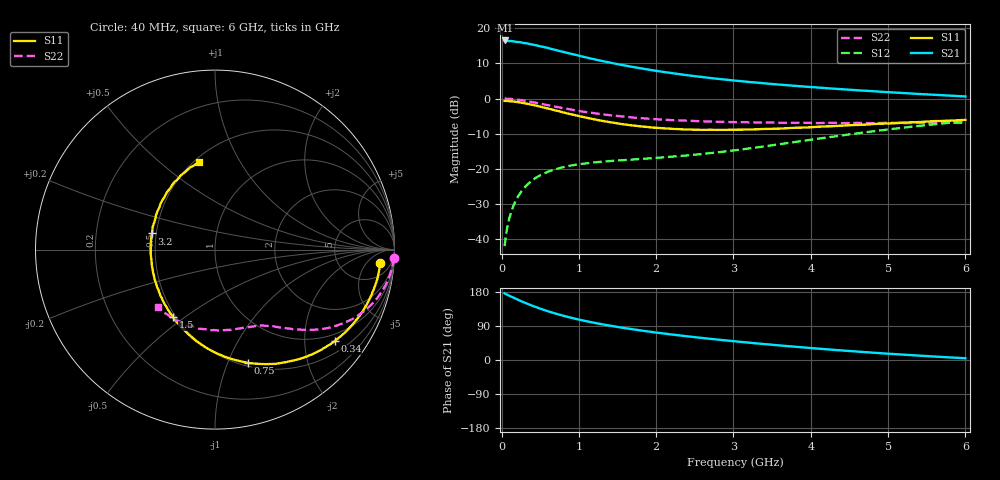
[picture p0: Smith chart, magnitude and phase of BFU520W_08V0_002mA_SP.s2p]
! Filename:  P:\Prog\Test\Noise\ATS_data\Testdata_Net\Run2\BFU520W_APM2013_06_A05_08p0V_002mA_SP_CM01_D.s2p
! Date/Time: Tue 26/Mar/2013 18:01:42
! BFU520W_APM2013_06_A05_08p0V_1to20mA_SP_CM01_Bias2_R.s2p
! MDIF S-parameter v. bias file
! BFU520W_APM2013_06_A05_08p0V_1to20mA_SP_CM01
! Date/time Thu Mar 21 15:28:29 2013
! VAR V_out= 8.0000
! VAR I_out= 2.0000
! VAR V_in= 0.8065
! VAR I_in= 0.0215
! Device data file deembeded for feedlines and parallel
! Original file: \Run2\BFU520W_APM2013_06_A05_08p0V_002mA_SP_CM01_R.s2p
! Feed-files: PR019V01_070313_Feed1.s2p, PR019V01_070313_Feed2.s2p
! Parallel-file: PR019V01_070313_Par.s2p
# MHz S MA R 50
!  Freq-MHz  S11-mag  S11-arg  S21-mag  S21-arg  S12-mag  S12-arg  S22-mag  S22-arg
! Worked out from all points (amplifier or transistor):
!   98 points, 40 MHz to 6 GHz, reference 50 ohm
!   highest |S21| = 16.5 dB at 50 MHz (marker M1)
!   |S21| within 3 dB of that: start of sweep to 750.4 MHz
!   unconditionally stable (mu >= 1): 2.391 GHz to 3.471 GHz
!   at 300 MHz: K = 0.18, MSG = 20.5 dB, |S12| = -25.2 dB
!   at 1.6 GHz: K = 0.78, MSG = 13.4 dB, |S12| = -17.5 dB
!   at 6 GHz: K = 0.82, MSG = 3.5 dB, |S12| = -6.5 dB
!   S11 on the Smith chart (normalised r, x): 40 MHz: 12, -13; 340 MHz: 0.79, -2.74; 750 MHz: 0.53, -1.18; 1.5 GHz: 0.48, -0.45; 3.2 GHz: 0.47, +0.10; 6 GHz: 0.53, +0.69
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40  0.9244 -4.6  6.654 176.0  0.00799 86.8  0.9968 -2.6
50  0.9233 -5.7  6.678 174.8  0.009908 86.3  0.9951 -3.2
90  0.9189 -10.3  6.546 170.7  0.01775 83.5  0.9912 -5.9
120  0.9124 -13.8  6.574 167.8  0.02349 81.4  0.986 -7.8
220  0.8853 -24.8  6.356 158.4  0.04164 75.0  0.9585 -13.9
340  0.8396 -37.5  6.038 147.9  0.06068 68.1  0.9138 -20.6
420  0.8038 -45.3  5.785 141.5  0.07162 64.1  0.8806 -24.4
550  0.7428 -57.5  5.375 132.0  0.08619 58.5  0.8241 -29.8
600  0.7213 -61.9  5.227 128.7  0.09104 56.6  0.8036 -31.6
750  0.6566 -73.9  4.728 119.6  0.1028 52.1  0.7461 -36.3
900  0.5973 -85.1  4.314 111.5  0.1118 48.7  0.697 -40.0
1050  0.5482 -95.3  3.933 104.5  0.1182 46.4  0.6524 -43.1
1250  0.4932 -107.7  3.508 96.2  0.1253 44.4  0.6079 -46.5
1500  0.4432 -121.8  3.079 87.2  0.1316 43.6  0.5642 -50.2
1800  0.4018 -137.3  2.686 78.0  0.1384 44.3  0.5258 -54.0
2050  0.3806 -149.1  2.424 71.2  0.1446 45.7  0.5042 -57.1
2500  0.3599 -168.7  2.079 60.2  0.1592 49.2  0.4792 -63.2
3100  0.3614 169.0  1.76 47.7  0.1889 54.3  0.4611 -72.4
3200  0.3624 165.6  1.719 45.8  0.1954 54.9  0.4583 -73.9
4100  0.3974 139.8  1.431 29.9  0.2691 56.9  0.4483 -90.9
5200  0.4549 115.0  1.196 14.1  0.3856 50.8  0.4465 -115.0
6000  0.4975 100.0  1.07 4.6  0.4739 43.0  0.4491 -134.9
